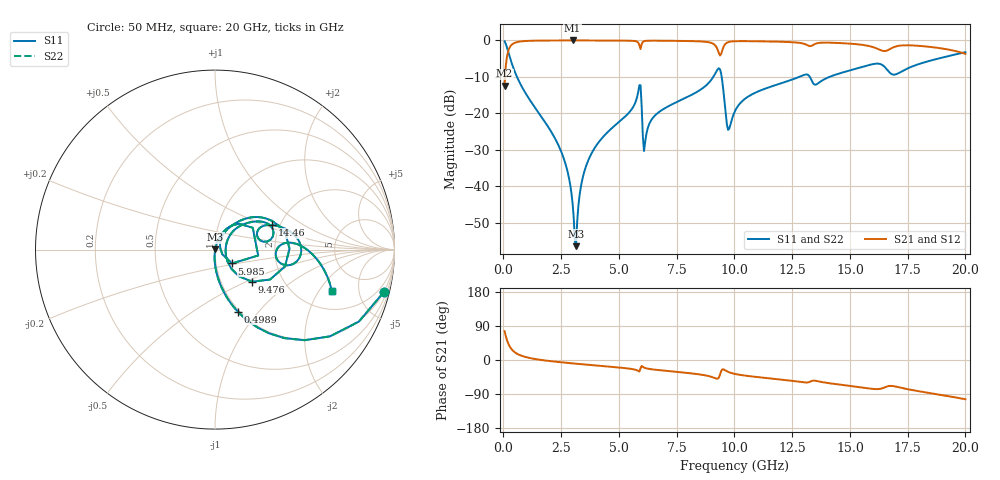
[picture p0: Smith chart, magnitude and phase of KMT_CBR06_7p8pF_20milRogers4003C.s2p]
! Data measured by Modelithics Inc. support@modelithics.com 813-866-6335
! KEMET CBR0603 7.8pF, Pad Width= 0.851mm, Pad Length= 0.64mm, Pad Gap= 0.62mm, 20mil Rogers 4003C substrate Data, January 2022
# hz S ma R 50
! 2 Port Network Data from SP1.SP block
! freq  magS11  angS11  magS21  angS21  magS12  angS12  magS22  angS22
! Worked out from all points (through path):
!   401 points, 50 MHz to 20 GHz, reference 50 ohm
!   highest |S21| = -0.01 dB at 2.993 GHz (marker M1); lowest = -12.4 dB at 50 MHz (marker M2)
!   group delay of S21, straight-line fit = 14.8 ps
!   lowest |S11| = -56.4 dB at 3.142 GHz (marker M3), VSWR 1.00, Z = 50.1 + j0.0654 ohm
!   |S11| at or under -10 dB: 586.5 MHz to 9.086 GHz (8.499 GHz wide, 176 % of centre); 9.447 GHz to 12.8 GHz (3.357 GHz wide, 30.2 % of centre); 13.27 GHz to 14.12 GHz (851.6 MHz wide, 6.22 % of centre)
!   |S22| runs from -56.4 to -0.3 dB; largest |S21 - S12| = 0
!   S11 on the Smith chart (normalised r, x): 50 MHz: 0.98, -8.01; 498.9 MHz: 0.98, -0.78; 5.985 GHz: 1.19, -0.19; 9.476 GHz: 1.40, -0.54; 14.46 GHz: 1.82, +0.57; 20 GHz: 2.99, -2.63
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5e7  0.9707 -14.0  0.2399 75.9  0.2399 75.9  0.9707 -14.0
2.495e8  0.6273 -51.9  0.778 38.1  0.778 38.1  0.6273 -51.9
4.98875e8  0.3677 -69.9  0.9291 20.0  0.9291 20.0  0.3677 -69.9
2.444e9  0.03295 -93.8  0.9983 -5.7  0.9983 -5.7  0.03295 -93.8
2.793125e9  0.01505 -93.4  0.9986 -7.8  0.9986 -7.8  0.01505 -93.4
2.992625e9  0.005859 -87.1  0.9987 -9.0  0.9987 -9.0  0.005859 -87.1
3.14225e9  0.001508 25.6  0.9987 -9.8  0.9987 -9.8  0.001508 25.6
3.391625e9  0.01146 72.4  0.9985 -11.2  0.9985 -11.2  0.01146 72.4
3.94025e9  0.03313 73.5  0.9979 -14.1  0.9979 -14.1  0.03313 73.5
5.8355e9  0.1969 47.0  0.9337 -29.0  0.9337 -29.0  0.1969 47.0
5.985125e9  0.1222 -39.1  0.8864 -15.7  0.8864 -15.7  0.1222 -39.1
6.13475e9  0.04008 46.0  0.9835 -21.1  0.9835 -21.1  0.04008 46.0
6.73325e9  0.1041 61.5  0.9911 -26.7  0.9911 -26.7  0.1041 61.5
9.077375e9  0.3131 35.0  0.9013 -45.9  0.9013 -45.9  0.3131 35.0
9.476375e9  0.2732 -40.9  0.7344 -24.7  0.7344 -24.7  0.2732 -40.9
9.72575e9  0.05941 -7.1  0.9451 -31.2  0.9451 -31.2  0.05941 -7.1
1.0025e10  0.1073 42.6  0.9742 -36.8  0.9742 -36.8  0.1073 42.6
1.336662e10  0.2718 9.3  0.8507 -54.9  0.8507 -54.9  0.2718 9.3
1.446388e10  0.3458 23.3  0.9229 -64.2  0.9229 -64.2  0.3458 23.3
1.670825e10  0.3657 -11.2  0.7533 -68.5  0.7533 -68.5  0.3657 -11.2
1.790525e10  0.4646 3.5  0.846 -81.6  0.846 -81.6  0.4646 3.5
2e10  0.6902 -19.5  0.6538 -103.5  0.6538 -103.5  0.6902 -19.5
